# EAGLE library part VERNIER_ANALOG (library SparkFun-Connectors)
British Telecom Connector - BTA (female) This device is useful when designing a project that uses any of the analog sensors in the Vernier ecosystem (sensors and/or controllers) SparkFun Products: SparkFun Vernier Interface Shield (DEV-12858) British Telecom Connector - BTA (female)
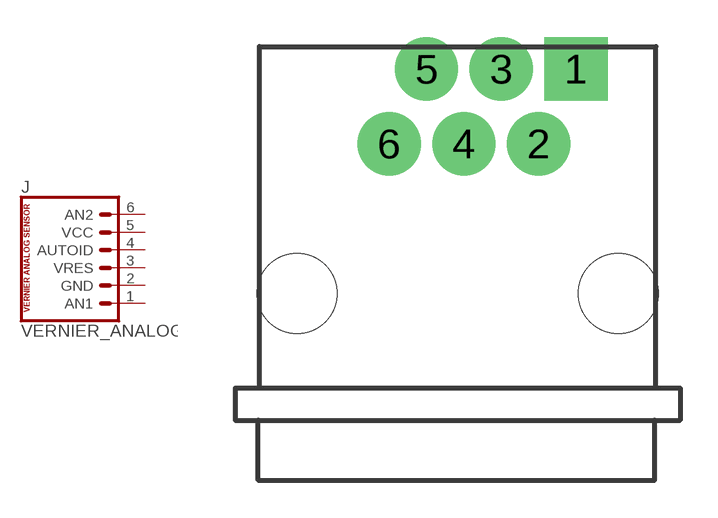
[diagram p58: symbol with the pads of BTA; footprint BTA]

Designator prefix J

## VERNIER_ANALOG (PROD_ID: CONN-11653; SF_ID: PRT-12753)  [BTA]
1  AN1  pas
2  GND  pas
3  VRES  pas
4  AUTOID  pas
5  VCC  pas
6  AN2  pas

## Footprint BTA (pad centres in mm)
British Telecom Connector - Analog Right Angle Specifications: Pin count: 6 Datasheet referenced for footprint Example device(s): VERNIER_ANALOG
drill 1.4 pad 2.54 square: 1 4.75,9
drill 1.4 pad 2.54: 2 3.25,6; 3 1.75,9; 4 0.25,6; 5 -1.25,9; 6 -2.75,6
hole 3.2 at 6.45,0
hole 3.2 at -6.45,0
